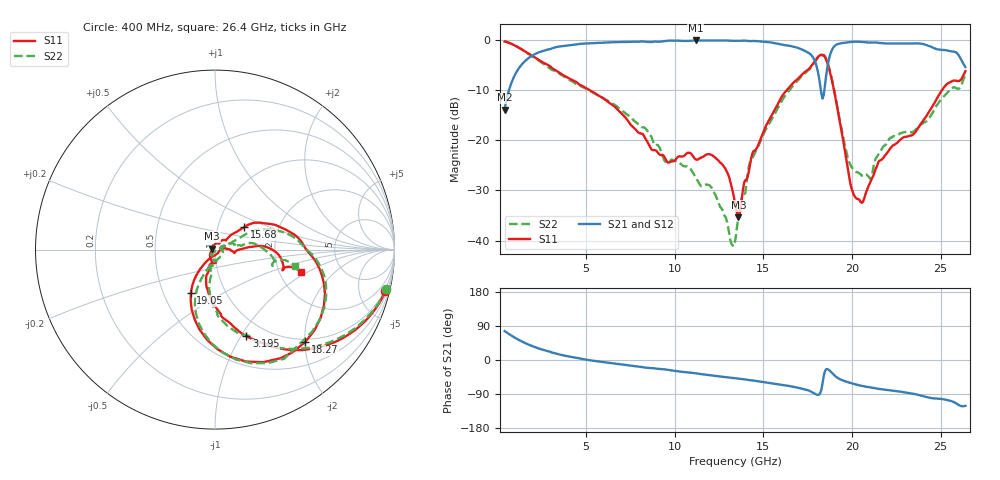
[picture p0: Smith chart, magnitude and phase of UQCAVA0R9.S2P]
!  Part Number  UQCAVA0R9
!  Description: RF capacitor  Mounting Orientation: Horizontal
!  Application:
# GHZ S DB R 50
! Freq  |S11|  S11 Ph  |S21|  S21 Ph  |S12|  S12 Ph  |S22|  S22 Ph
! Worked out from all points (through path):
!   401 points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, 400 MHz to 26.4 GHz, reference 50 ohm
!   highest |S21| = -0.01 dB at 11.19 GHz (marker M1); lowest = -13.8 dB at 400 MHz (marker M2)
!   lowest |S11| = -35.4 dB at 13.6 GHz (marker M3), VSWR 1.03, Z = 48.4 + j0.566 ohm
!   |S11| at or under -10 dB: 5.238 GHz to 16.31 GHz (11.07 GHz wide, 103 % of centre); 18.99 GHz to 25.07 GHz (6.076 GHz wide, 27.6 % of centre)
!   |S22| runs from -41.1 to -0.2 dB; largest |S21 - S12| = 0.0031
!   S11 on the Smith chart (normalised r, x): 400 MHz: 0.80, -8.24; 3.195 GHz: 0.80, -1.06; 15.68 GHz: 1.34, +0.35; 18.27 GHz: 0.94, -2.01; 19.05 GHz: 0.69, -0.36; 26.4 GHz: 2.63, -0.85
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0.4  -0.20 -13.7  -13.83 76.4  -13.84 76.4  -0.19 -13.1
1.375  -1.80 -41.3  -4.78 48.8  -4.79 48.8  -1.84 -40.3
3.195  -5.79 -70.1  -1.45 18.4  -1.46 18.4  -6.03 -71.8
4.755  -9.04 -85.6  -0.67 2.9  -0.67 3.0  -9.23 -88.8
9.11  -22.71 -101.4  -0.27 -23.4  -0.26 -23.4  -21.22 -99.8
11.19  -23.79 -95.2  -0.01 -35.2  -0.01 -35.2  -27.46 -118.9
12.62  -24.55 -112.8  -0.03 -43.8  -0.03 -43.9  -33.49 -122.8
13.4  -32.48 -157.7  -0.08 -48.2  -0.08 -48.2  -40.17 -30.1
13.595  -35.38 159.9  -0.09 -49.2  -0.08 -49.2  -35.41 -3.6
14.31  -23.61 52.6  -0.13 -53.4  -0.13 -53.5  -23.85 17.3
15.675  -13.69 37.5  -0.57 -63.5  -0.57 -63.5  -14.45 26.6
17.755  -4.88 -7.4  -3.16 -85.1  -3.15 -85.1  -5.08 -4.6
18.275  -2.86 -45.7  -10.65 -78.1  -10.65 -78.1  -2.99 -40.4
18.535  -3.78 -74.5  -7.27 -24.6  -7.26 -24.6  -3.55 -72.3
19.055  -11.19 -119.2  -1.00 -42.5  -0.99 -42.6  -11.07 -112.9
19.77  -25.71 -118.2  -0.37 -58.5  -0.37 -58.6  -23.53 -91.4
20.225  -31.52 -65.9  -0.26 -64.6  -0.26 -64.7  -26.29 -52.9
21.005  -28.58 1.1  -0.44 -71.9  -0.44 -72.0  -27.58 -3.0
22.11  -21.88 1.1  -0.64 -79.6  -0.63 -79.7  -19.68 20.1
23.995  -16.16 2.0  -0.71 -95.2  -0.71 -95.4  -16.56 8.4
25.75  -8.03 -15.1  -2.25 -110.9  -2.25 -111.1  -9.37 -13.4
26.4  -6.14 -14.4  -5.32 -121.1  -5.31 -121.2  -6.80 -11.4
